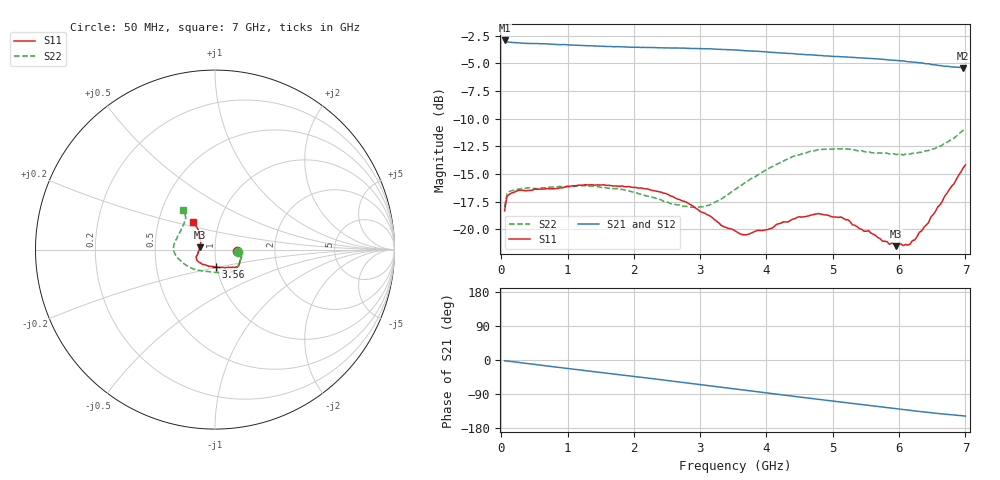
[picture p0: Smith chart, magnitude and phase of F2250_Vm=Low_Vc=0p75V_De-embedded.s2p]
! Integrated Device Technology
! Corporate Headquarters
! 6024 Silver Creek Valley Road
! San Jose, CA 95138  USA
! Phone:  1-408-284-8200
! Toll Free:  1-800-223-1366
! Webpage:  http://www.idt.com/
! Timing and RF Division
! 515 Groton Road, Suite 102
! Westford, MA 01886-6024
! Device:  F2250
! Description: Voltage Variable RF Attenuator
! Frequency:  50.0 -  6000.00 MHz
! Package:  3x3 mm Thin QFN Plastic Package: 16 pin
! Ports:  2 RF, 3 DC
!  Pin  1  = GND
!  Pin  2  = NC
!  Pin  3  = RF1  = Port 1
!  Pin  4  = NC
!  Pin  5  = GND
!  Pin  6  = GND
!  Pin  7  = GND
!  Pin  8  = GND
!  Pin  9  = NC
!  Pin 10  = RF2  = Port 2
!  Pin 11  = NC
!  Pin 12  = GND
!  Pin 13  = GND
!  Pin 14  = VCNTRL
!  Pin 15  = VDD
!  Pin 16  = VMODE
! Vcntrl:  0.750 Volts
! Vmode:  +0.000 Volts
! Vdd:  +3.30  Volts
! Current:  1.156 mA
! Data:  The device was measured on a the F2250 evaluation board which has
!  individual transmission lines to the RF pins.  Data was collected
!  using a calibrated network analyzer.  The evaluation board was
!  de-embedded using a TRL calibration technique.
!  The reference plane is the edge of the package pin.
! Misc:  SN 10
!  Action Tracker AT0258
! Date Measured:  2014-11-26
! Date:  2015-10-15  MJV
! Note:
!  Integrated Device Technology supplies this data as a sample of measured
!  data at the package pin for this product.  Your particular data for this
!  product may vary.
!  Data was taken at 25 degrees C.
!  Integrated Device Technology reserves the right to change this data at anytime.
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# GHz S dB R 50
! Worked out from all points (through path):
!   201 points, 50 MHz to 7 GHz, reference 50 ohm
!   highest |S21| = -2.92 dB at 50 MHz (marker M1); lowest = -5.4 dB at 6.965 GHz (marker M2)
!   group delay of S21, straight-line fit = 59.3 ps
!   lowest |S11| = -21.5 dB at 5.957 GHz (marker M3), VSWR 1.18, Z = 42.3 + j1.03 ohm
!   |S11| at or under -10 dB: start of sweep to end of sweep
!   |S22| runs from -18.0 to -10.9 dB; largest |S21 - S12| = 0.0015
!   S11 on the Smith chart (normalised r, x): 50 MHz: 1.27, -0.03; 3.56 GHz: 0.99, -0.19; 7 GHz: 0.75, +0.24
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0.05  -18.32 -4.7  -2.92 -2.1  -2.93 -2.1  -17.98 -5.9
0.08475  -17.06 -4.1  -3.05 -2.6  -3.04 -2.6  -16.81 -5.3
0.22375  -16.55 -7.3  -3.13 -5.6  -3.13 -5.6  -16.40 -9.8
0.6755  -16.33 -19.5  -3.22 -15.4  -3.24 -15.4  -16.23 -26.3
1.2315  -16.00 -32.2  -3.38 -27.3  -3.39 -27.3  -16.05 -45.5
1.82225  -16.08 -38.2  -3.50 -39.6  -3.50 -39.6  -16.39 -58.7
2.37825  -16.59 -41.8  -3.58 -51.3  -3.58 -51.3  -17.28 -71.6
2.7605  -17.47 -48.0  -3.61 -59.6  -3.63 -59.6  -17.93 -86.8
3.0385  -18.49 -57.0  -3.66 -65.7  -3.67 -65.7  -17.96 -102.8
3.525  -20.14 -84.9  -3.78 -76.5  -3.78 -76.5  -16.41 -131.5
3.55975  -20.26 -87.3  -3.78 -77.2  -3.79 -77.2  -16.25 -133.1
3.69875  -20.49 -98.4  -3.85 -80.3  -3.84 -80.3  -15.70 -140.0
4.39375  -19.08 -138.3  -4.10 -95.4  -4.11 -95.4  -13.43 -167.1
4.7065  -18.67 -148.8  -4.23 -102.2  -4.24 -102.2  -12.92 -175.0
5.1235  -18.88 -158.2  -4.39 -111.0  -4.39 -111.0  -12.73 175.3
5.85325  -21.35 178.1  -4.68 -126.2  -4.68 -126.3  -13.19 157.5
5.9575  -21.52 171.7  -4.72 -128.4  -4.72 -128.5  -13.24 154.6
6.13125  -21.42 160.3  -4.84 -132.1  -4.83 -132.1  -13.19 148.7
6.2355  -20.96 151.7  -4.89 -134.3  -4.90 -134.3  -13.15 145.3
6.61775  -17.79 132.7  -5.19 -141.6  -5.20 -141.6  -12.49 133.4
6.96525  -14.46 128.2  -5.41 -147.4  -5.42 -147.4  -11.04 129.8
7  -14.17 127.8  -5.41 -147.9  -5.42 -147.9  -10.88 129.1
